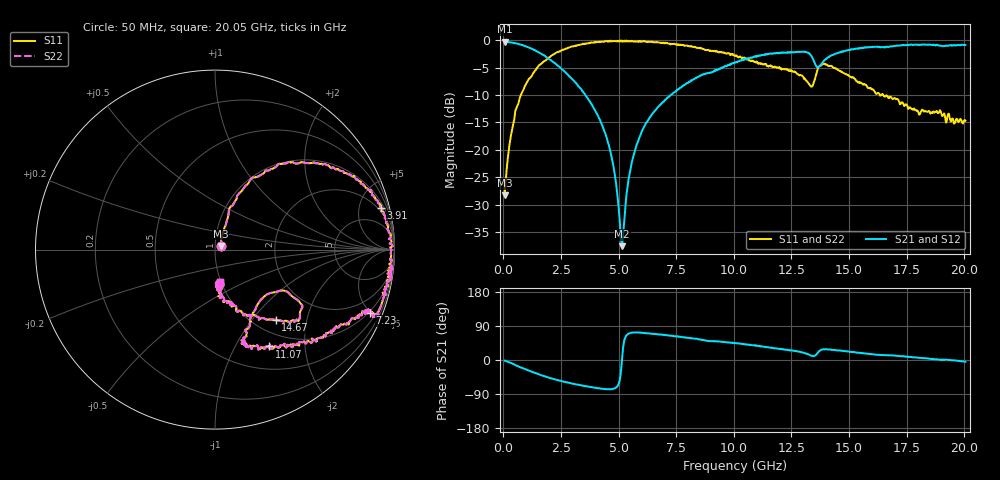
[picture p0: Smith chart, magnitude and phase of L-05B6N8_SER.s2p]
! P/N: L-05C6N8_SER
! Measured by Marlon
! Sep. 23, 2003
! Measure with a Series-through-fixture
#	mhz	s	ma	r	50
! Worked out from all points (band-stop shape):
!   1001 points, 50 MHz to 20.05 GHz, reference 50 ohm
!   highest |S21| = -0.27 dB at 70 MHz (marker M1); lowest = -37.5 dB at 5.15 GHz (marker M2)
!   |S21| within 3 dB of the highest: 10.65 GHz to 13.42 GHz (2.765 GHz wide, 23 % of centre); 14.04 GHz to end of sweep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
!   lowest |S11| = -28.3 dB at 50 MHz (marker M3), VSWR 1.08, Z = 53.3 + j2.22 ohm
!   |S11| at or under -10 dB: start of sweep to 754.9 MHz; 16.33723 GHz to 16.3921 GHz (54.87 MHz wide, 0.335 % of centre); 16.49 GHz to end of sweep
!   |S22| runs from -28.3 to 0.0 dB; largest |S21 - S12| = 0
!   S11 on the Smith chart (normalised r, x): 50 MHz: 1.07, +0.04; 3.91 GHz: 1.48, +7.77; 7.23 GHz: 0.94, -4.92; 11.07 GHz: 0.79, -1.38; 14.67 GHz: 1.23, -1.33; 20.05 GHz: 0.99, -0.37
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50  0.03865 32.5  0.9689 -1.6  0.9689 -1.6  0.03865 32.5
70  0.04327 41.0  0.969 -1.8  0.969 -1.8  0.04327 41.0
470  0.1887 68.0  0.9447 -11.4  0.9447 -11.4  0.1887 68.0
1010  0.4099 63.5  0.8727 -25.9  0.8727 -25.9  0.4099 63.5
2050  0.716 42.2  0.6604 -47.9  0.6604 -47.9  0.716 42.2
3390  0.9167 21.3  0.3531 -67.2  0.3531 -67.2  0.9167 21.3
3910  0.9546 14.2  0.2433 -72.6  0.2433 -72.6  0.9546 14.2
4670  0.9786 0.7  0.09083 -77.2  0.09083 -77.2  0.9786 0.7
5150  0.9706 -6.9  0.01326 4.4  0.01326 4.4  0.9706 -6.9
5430  0.9862 -10.3  0.05401 69.5  0.05401 69.5  0.9862 -10.3
5690  0.9748 -12.6  0.09653 72.8  0.09653 72.8  0.9748 -12.6
6110  0.9811 -21.6  0.1638 71.0  0.1638 71.0  0.9811 -21.6
6730  0.9578 -22.6  0.2488 67.3  0.2488 67.3  0.9578 -22.6
7230  0.9307 -22.2  0.3133 63.7  0.3133 63.7  0.9307 -22.2
10050  0.7208 -46.1  0.6256 44.1  0.6256 44.1  0.7208 -46.1
11070  0.6176 -60.9  0.7272 36.9  0.7272 36.9  0.6176 -60.9
12210  0.5437 -73.3  0.7717 27.6  0.7717 27.6  0.5437 -73.3
13390  0.3786 -43.5  0.7054 10.8  0.7054 10.8  0.3786 -43.5
13750  0.5842 -34.9  0.5863 25.4  0.5863 25.4  0.5842 -34.9
14670  0.5185 -49.3  0.7905 24.5  0.7905 24.5  0.5185 -49.3
16730  0.2964 -75.9  0.8693 12.0  0.8693 12.0  0.2964 -75.9
20050  0.1847 -81.0  0.9043 -4.6  0.9043 -4.6  0.1847 -81.0
